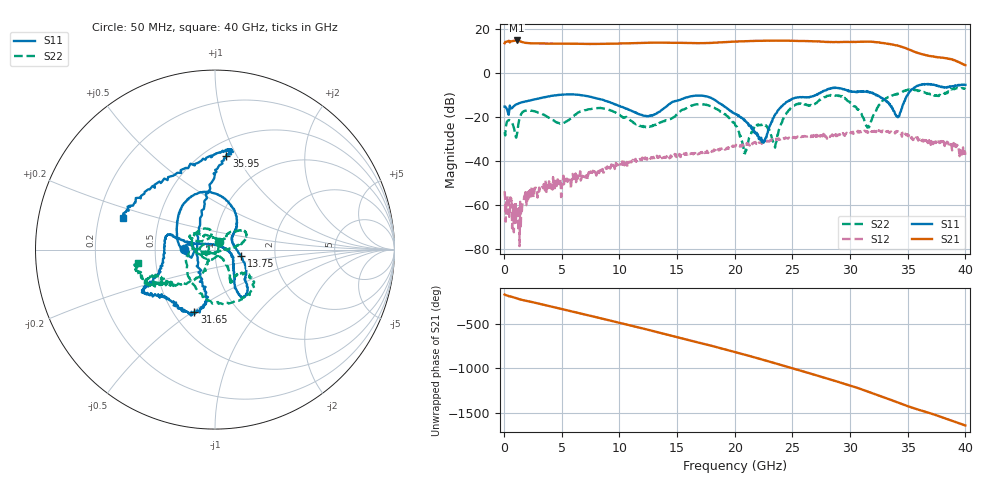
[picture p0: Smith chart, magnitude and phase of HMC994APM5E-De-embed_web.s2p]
! Analog Devices, Inc.
! Device:	HMC994APM5E
! Description:	GaAs PHEMT MMIC POWER AMPLIFIER, DC - 28 GHz
! Conditions:	Vdd = 10.0 V
!		Vgg2 = 3.5 V
!		Vgg1 = -0.5 V
!		Idd = 250 mA quiescent
!		Pin = -15 dBm
!		Operating Temperature = +25 C (at package bottom)
! This measurement was fully de-embedded to the input and output pins of the device.
! Frequency (GHz)	S11_Mag (dB)	S11_Phase (deg)	S21_Mag (dB)	S21_Phase (deg)	S12_Mag (dB)	S12_Phase (deg)	S22_Mag (dB)	S22_Phase (deg)
# Hz S  dB  R 50
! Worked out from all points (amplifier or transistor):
!   800 points, 50 MHz to 40 GHz, reference 50 ohm
!   highest |S21| = 14.9 dB at 1.1 GHz (marker M1)
!   |S21| within 3 dB of that: start of sweep to 34.55 GHz
!   unconditionally stable (mu >= 1): start of sweep to end of sweep
!   at 6.7 GHz: K = 24.49, MAG = 13.9 dB, |S12| = -48.2 dB
!   at 20.05 GHz: K = 4.45, MAG = 14.5 dB, |S12| = -33.4 dB
!   at 40 GHz: K = 13.66, MAG = 6.0 dB, |S12| = -37.2 dB
!   S11 on the Smith chart (normalised r, x): 50 MHz: 0.71, +0.01; 13.75 GHz: 1.34, -0.10; 31.65 GHz: 0.63, -0.51; 35.95 GHz: 0.63, +0.91; 40 GHz: 0.31, +0.15
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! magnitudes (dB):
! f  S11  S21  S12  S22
! 50 MHz  -15.3  13.7  -53.8  -26.9
! 450 MHz  -17.2  14.7  -65.5  -21.3
! 1.1 GHz  -14.1  14.9  -61.2  -28.5
! 1.85 GHz  -12.9  13.8  -54.3  -17.1
! 4.95 GHz  -9.8  13.4  -56.5  -22.9
! 6.75 GHz  -10.1  13.4  -46.7  -17.2
! 13.4 GHz  -17.8  13.9  -38.2  -23.2
! 13.75 GHz  -16.5  13.9  -38.5  -22.0
! 17.1 GHz  -10.2  13.7  -36.4  -14.2
! 20.05 GHz  -18.5  14.4  -33.4  -23.8
! 20.9 GHz  -21.8  14.5  -32.7  -36.6
! 21.75 GHz  -26.7  14.7  -31.8  -24.7
! 22.55 GHz  -30.8  14.8  -31.4  -23.6
! 23.45 GHz  -19.3  14.8  -30.2  -32.7
! 24.85 GHz  -12.1  14.7  -29.4  -16.0
! 26.7 GHz  -10.6  14.5  -29.0  -14.6
! 29.25 GHz  -7.0  14.2  -27.9  -10.6
! 31.65 GHz  -8.7  14.3  -26.4  -24.7
! 33.35 GHz  -13.5  13.3  -27.0  -10.8
! 34.2 GHz  -19.7  12.4  -26.8  -9.2
! 35.95 GHz  -5.6  9.1  -30.4  -8.1
! 40 GHz  -5.3  3.6  -37.2  -7.3
